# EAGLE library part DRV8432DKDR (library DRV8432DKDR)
12A Dual Brushed DC or Single Bipolar Stepper Motor Driver (PWM Ctrl) Source: Datasheet
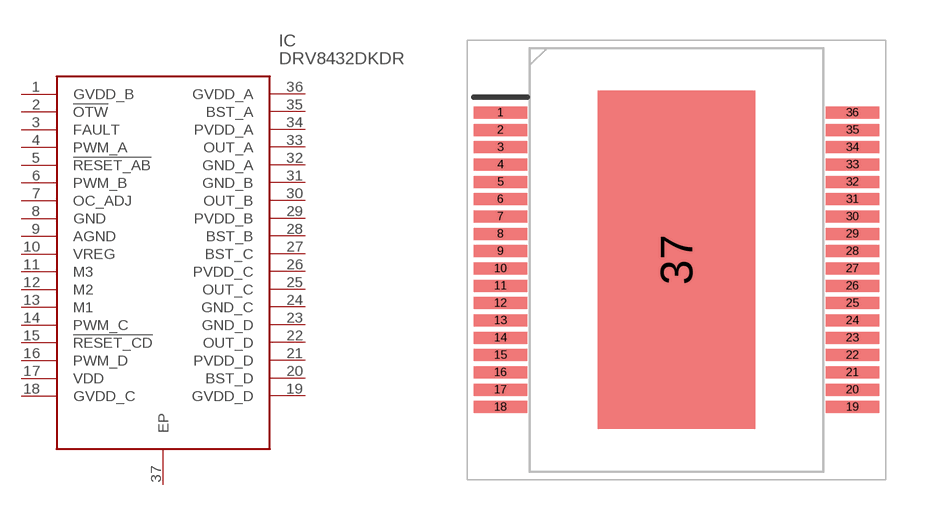
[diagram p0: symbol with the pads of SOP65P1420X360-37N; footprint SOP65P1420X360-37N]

Designator prefix IC

## DRV8432DKDR (Description: 12A Dual Brushed DC or Single Bipolar Stepper Motor Driver (PWM Ctrl); Height: 3.6mm; Manufacturer_Name: Texas Instruments; Manufacturer_Part_Number: DRV8432DKDR; Mouser_Part_Number: 595-DRV8432DKDR; Mouser_Price-Stock: https://www.mouser.com/Search/Refine.aspx?Keyword=595-DRV8432DKDR)  [SOP65P1420X360-37N]
1  GVDD_B
2  !OTW
3  FAULT
4  PWM_A
5  !RESET_AB
6  PWM_B
7  OC_ADJ
8  GND
9  AGND
10  VREG
11  M3
12  M2
13  M1
14  PWM_C
15  !RESET_CD
16  PWM_D
17  VDD
18  GVDD_C
19  GVDD_D
20  BST_D
21  PVDD_D
22  OUT_D
23  GND_D
24  GND_C
25  OUT_C
26  PVDD_C
27  BST_C
28  BST_B
29  PVDD_B
30  OUT_B
31  GND_B
32  GND_A
33  OUT_A
34  PVDD_A
35  BST_A
36  GVDD_A
37  EP

## Footprint SOP65P1420X360-37N (pad centres in mm)
DKD (R-PDSO-G36)
smd 2 x 0.45: 1 -6.6,5.525; 2 -6.6,4.875; 3 -6.6,4.225; 4 -6.6,3.575; 5 -6.6,2.925; 6 -6.6,2.275; 7 -6.6,1.625; 8 -6.6,0.975; 9 -6.6,0.325; 10 -6.6,-0.325; 11 -6.6,-0.975; 12 -6.6,-1.625; 13 -6.6,-2.275; 14 -6.6,-2.925; 15 -6.6,-3.575; 16 -6.6,-4.225; 17 -6.6,-4.875; 18 -6.6,-5.525; 19 6.6,-5.525; 20 6.6,-4.875; 21 6.6,-4.225; 22 6.6,-3.575; 23 6.6,-2.925; 24 6.6,-2.275; 25 6.6,-1.625; 26 6.6,-0.975; 27 6.6,-0.325; 28 6.6,0.325; 29 6.6,0.975; 30 6.6,1.625; 31 6.6,2.275; 32 6.6,2.925; 33 6.6,3.575; 34 6.6,4.225; 35 6.6,4.875; 36 6.6,5.525
smd 5.9 x 12.7: 37 0,0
